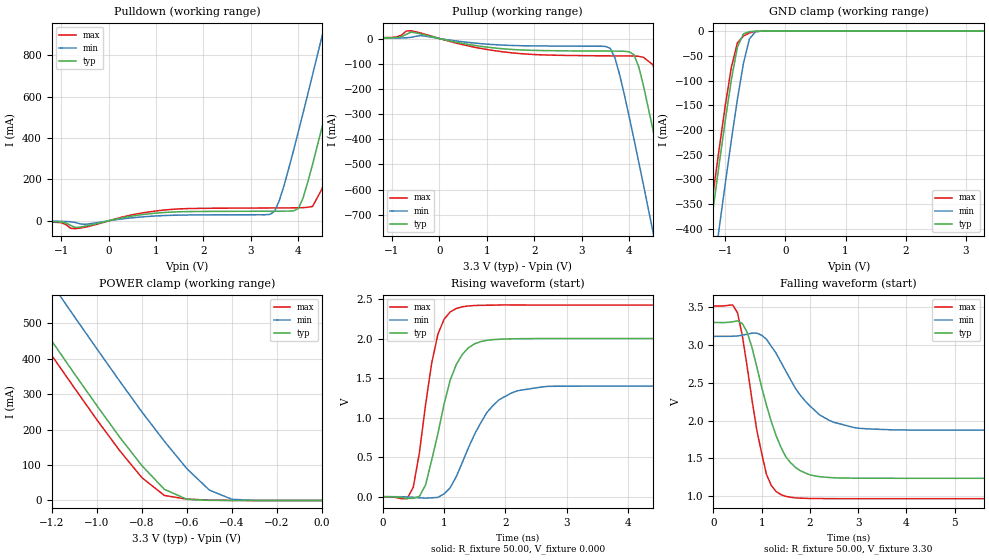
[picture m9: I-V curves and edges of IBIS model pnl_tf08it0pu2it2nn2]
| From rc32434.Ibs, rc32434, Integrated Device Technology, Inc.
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[Model]   pnl_tf08it0pu2it2nn2
Model_type   I/O
Polarity   Non-Inverting
Enable   Active-High
Vinl =  0.800V
Vinh =  2.000V
Vmeas =  1.500V
C_comp   0.40pF   0.30pF   0.50pF
[Temperature Range]   25.00   0.12k   0.000
[Voltage Range]   3.30V   3.00V   3.60V
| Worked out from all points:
|   slope of the pulldown table from 0 to 0.495 V, typ, clamps not added: 21.5 ohm
|   slope of the pullup table from 0 to 0.495 V, typ, clamps not added: 25.2 ohm
|   GND clamp passes 1 mA (typ) near -0.59 V on its own axis
|   POWER clamp passes 1 mA (typ) near -0.52 V on its own axis
|   rising waveform, R_fixture 50.00, V_fixture 0.000: 20-80 % time 384ps typ, 545ps min, 285ps max; typ from 0 V to 2 V
|   falling waveform, R_fixture 50.00, V_fixture 3.30: 20-80 % time 567ps typ, 802ps min, 404ps max; typ from 3.3 V to 1.24 V
[Pulldown]
| voltage   I(typ)   I(min)   I(max)
-3.3V     -1mA       -1mA       -1mA
-700mV    -32.15mA   -8.02mA    -37.86mA
1.1V      39.14mA    24.71mA    50.34mA
3.4V      46.43mA    31.06mA    62.07mA
3.6V      46.61mA    98.81mA    62.29mA
4V        59.38mA    431mA      63.06mA
4.3V      273mA      706mA      69.58mA
4.5V      453mA      892mA      155mA
4.9V      827mA      1.264A     506mA
5.1V      1.015A     1.45A      693mA
5.3V      1.203A     1.636A     882mA
6.6V      2.429A     2.849A     2.111A
[Pullup]
| voltage   I(typ)   I(min)   I(max)
-3.3V     1mA        1mA        1mA
-1V       2.9mA      1.3mA      4.4mA
-600mV    25.38mA    4.68mA     30.91mA
1.3V      -40.12mA   -25.86mA   -51.88mA
3.6V      -50mA      -38.84mA   -68.88mA
3.8V      -50.18mA   -145mA     -69.1mA
4.1V      -63.99mA   -399mA     -69.5mA
4.3V      -187mA     -581mA     -74.65mA
4.5V      -361mA     -767mA     -104mA
4.9V      -732mA     -1.142A    -422mA
5.3V      -1.11A     -1.517A    -795mA
6.6V      -2.343A    -2.738A    -2.031A
[GND_clamp]
| voltage   I(typ)   I(min)   I(max)
-3.3V     -2.341A    -2.454A    -2.313A
-1.3V     -448mA     -579mA     -416mA
-1.2V     -356mA     -487mA     -324mA
-1.1V     -266mA     -396mA     -235mA
-1V       -179mA     -307mA     -149mA
-900mV    -97.89mA   -220mA     -72.81mA
-800mV    -32.55mA   -138mA     -23.92mA
-700mV    -5.649mA   -65.57mA   -9.936mA
-600mV    -1.103mA   -15.75mA   -3.555mA
-500mV    -147uA     -1.348mA   -664uA
-300mV    -14.87uA   -13.41uA   -23.57uA
3.3V      3.492nA    199uA      4.709nA
[POWER_clamp]
| voltage   I(typ)   I(min)   I(max)
-3.3V     2.427A     2.567A     2.391A
-1.4V     636mA      797mA      595mA
-1.3V     542mA      704mA      502mA
-1.2V     450mA      611mA      409mA
-1.1V     358mA      519mA      318mA
-900mV    180mA      338mA      142mA
-800mV    98.49mA    250mA      64.55mA
-700mV    31.46mA    167mA      14.17mA
-600mV    3.328mA    89.59mA    3.832mA
-500mV    386uA      29.21mA    1.198mA
-400mV    40.59uA    3.369mA    173uA
0V        3.492nA    3.771nA    1.445nA
[Ramp]
| variable   typ   min   max
dV/dt_r   1.20/0.38n   0.84/0.55n   1.46/0.28n
dV/dt_f   1.24/0.57n   0.84/0.81n   1.50/0.43n
R_load = 50.00
[Rising Waveform]
R_fixture = 50.00
V_fixture = 0.000
| time   V(typ)   V(min)   V(max)
0s        174uV      143uV      214uV
400ps     -21.05mV   -2.553mV   -25.03mV
500ps     -20.91mV   -7.532mV   120mV
700ps     148mV      -17.69mV   1.164V
900ps     795mV      -8.414mV   2.054V
1.1ns     1.474V     113mV      2.34V
1.2ns     1.674V     254mV      2.384V
1.7ns     1.981V     1.069V     2.425V
2.2ns     2.001V     1.343V     2.428V
9.9ns     2.003V     1.401V     2.427V
[Falling Waveform]
R_fixture = 50.00
V_fixture = 3.30
| time   V(typ)   V(min)   V(max)
0s        3.3V       3.117V     3.519V
500ps     3.322V     3.122V     3.429V
700ps     3.172V     3.145V     2.714V
900ps     2.712V     3.159V     1.873V
1.1ns     2.203V     3.078V     1.287V
1.4ns     1.647V     2.775V     1.019V
1.7ns     1.381V     2.427V     977mV
2.2ns     1.258V     2.076V     968mV
3ns       1.238V     1.9V       966mV
9.9ns     1.236V     1.874V     966mV
